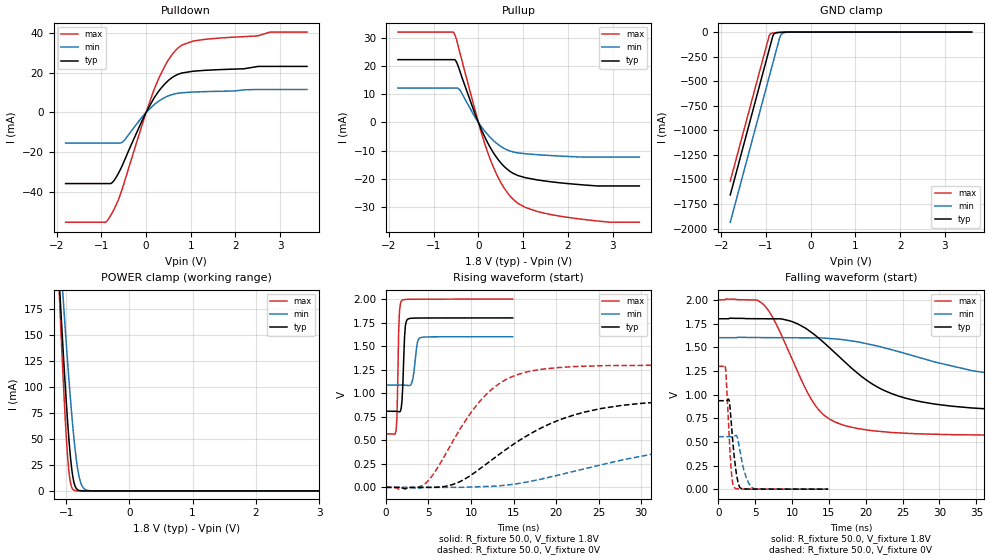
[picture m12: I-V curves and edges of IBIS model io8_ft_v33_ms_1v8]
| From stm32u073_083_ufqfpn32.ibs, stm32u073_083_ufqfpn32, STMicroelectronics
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[Model]   io8_ft_v33_ms_1v8
Model_type I/O
Polarity   Non-Inverting
Enable   Active-Low
| CAP_THRESHOLD on pad IOFT is "UDTCAPC" :
| Rising=30.0% of vddiom   Falling=70.0% of vddiom
| C_comp min and max val. don't necessarily correlate with the min and max pvt
| but are the smallest and greatest pad capacitance found.
| var   typ   min   max
C_comp   2.10717pF  2.10454pF  2.16860pF
|C_comp_pullup   1.19920pF  1.17990pF  1.18495pF
|C_comp_pulldown   907.97820fF  924.64068fF  983.64502fF
Vinl = 480.0mV
Vinh = 1.4V
Vmeas = 900.0mV   | Reference voltage for timing measurements
Cref  = 50.0pF   | Timing specification test load capacitance value
Rref  = 100.0MOhm   | Timing specification test load resistance value
Vref  = 900.0mV   | Timing specification test load voltage
[Model Spec]
| TIME_THRESHOLD on pin ZIV33M is "CMOS" :
| Rising=50.0% of vddiom   Falling=50.0% of vddiom
Vinl 728.70000mV 655.70000mV 817.70000mV
Vinh 1.06430V 949.30000mV 1.16330V
| variable   typ   min   max
[Temperature Range] 25.0 140.0 -40.0
| variable   typ   min   max
[Voltage Range] 1.8V 1.6V 2.0V
| variable   typ   min   max
[POWER Clamp Reference] 1.8V 1.6V 2.0V
| variable   typ   min   max
[GND Clamp Reference] 0V 0V 0V
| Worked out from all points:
|   slope of the pulldown table from 0 to 0.27 V, typ, clamps not added: 26.3 ohm
|   slope of the pullup table from 0 to 0.27 V, typ, clamps not added: 30 ohm
|   GND clamp passes 1 mA (typ) near -0.61 V on its own axis
|   POWER clamp passes 1 mA (typ) near -0.81 V on its own axis
|   rising waveform, R_fixture 50.0, V_fixture 1.8V: 20-80 % time 251ps typ, 394ps min, 200ps max; typ from 0.809 V to 1.8 V
|   falling waveform, R_fixture 50.0, V_fixture 1.8V: 20-80 % time 10.1ns typ, 18ns min, 5.4ns max; typ from 1.8 V to 0.809 V
|   rising waveform, R_fixture 50.0, V_fixture 0V: 20-80 % time 10.5ns typ, 18.9ns min, 5.99ns max; typ from 0 V to 0.935 V
|   falling waveform, R_fixture 50.0, V_fixture 0V: 20-80 % time 695ps typ, 1.01ns min, 535ps max; typ from 0.935 V to 0 V
[POWER Clamp]
-1.8V     1.053A     943.1mA    1.262A
-1.11V    202.2mA    242.3mA    190.9mA
-1.09V    180mA      223.6mA    163.4mA
-1.05V    136.9mA    187mA      110.9mA
-980mV    68.91mA    126.1mA    35.23mA
-940mV    37.57mA    94.11mA    10.65mA
-880mV    8.969mA    52.17mA    807.4uA
-830mV    1.697mA    25.82mA    75.79uA
-790mV    394.2uA    12.22mA    11.25uA
-740mV    61.25uA    3.879mA    1.034uA
-660mV    3.073uA    483.4uA    22.7nA
3.6V      0A         0A         0A
[GND Clamp]
-1.8V     -1.658A    -1.935A    -1.517A
-930mV    -179mA     -456mA     -38.91mA
-900mV    -128mA     -405mA     -17.65mA
-850mV    -44.09mA   -320mA     -9.519mA
-830mV    -24.74mA   -286mA     -8.302mA
-790mV    -9.695mA   -218mA     -6.49mA
-700mV    -2.938mA   -65mA      -3.294mA
-670mV    -2.157mA   -31.85mA   -2.435mA
-640mV    -1.545mA   -16.21mA   -1.699mA
-570mV    -571.9uA   -3.807mA   -536.5uA
-420mV    -14.26uA   -143.3uA   -5.434uA
3.6V      449.1pA    102.3nA    316.4pA
| variable   typ   min   max
[Pullup Reference] 1.8V 1.6V 2.0V
| variable   typ   min   max
[Pulldown Reference] 0V 0V 0V
[Pullup]
-1.8V     22.25mA    12.18mA    32.02mA
-550mV    22.25mA    12.18mA    31.76mA
-500mV    21.67mA    12.18mA    29.82mA
-420mV    18.45mA    11.57mA    25.1mA
-90mV     3.62mA     2.224mA    5.223mA
240mV     -8.143mA   -4.875mA   -12mA
540mV     -15mA      -8.867mA   -22.31mA
870mV     -18.72mA   -10.75mA   -28.48mA
1.33V     -20.4mA    -11.44mA   -31.6mA
1.9V      -21.5mA    -11.96mA   -33.39mA
2.94V     -22.49mA   -12.26mA   -35.33mA
3.6V      -22.49mA   -12.26mA   -35.33mA
[Pulldown]
-1.8V     -35.76mA   -15.41mA   -55.17mA
-910mV    -35.76mA   -15.41mA   -55.17mA
-830mV    -35.76mA   -15.41mA   -53.18mA
-710mV    -34mA      -15.41mA   -48.42mA
-520mV    -26.05mA   -14.75mA   -37.5mA
-90mV     -4.145mA   -2.306mA   -6.327mA
230mV     8.974mA    4.797mA    14.24mA
490mV     15.87mA    8.223mA    26.01mA
750mV     19.43mA    9.743mA    33.01mA
1.33V     21.16mA    10.45mA    36.75mA
2.78V     23.13mA    11.52mA    40.36mA
3.6V      23.13mA    11.52mA    40.37mA
[Ramp]
dV/dt_r 560.73538mV/10.49232ns 332.40859mV/18.92225ns 778.78175mV/5.99118ns
dV/dt_f 594.8441mV/10.08343ns 308.2854mV/17.96303ns 859.13306mV/5.40114ns
R_load = 50.0
| Removed startup time: 0s 0s 0s  .
| Removed end time: 14.9ns.
[Rising Waveform]
R_fixture   = 50.0
V_fixture   = 1.8V
V_fixture_min = 1.6V
V_fixture_max = 2.0V
0s        808.6mV    1.086V     568.1mV
1.2ns     808.3mV    1.086V     602.5mV
1.3ns     807.6mV    1.086V     728.9mV
1.5ns     803.8mV    1.086V     1.641V
1.6ns     801.6mV    1.086V     1.871V
1.9ns     923.4mV    1.086V     1.987V
2.2ns     1.607V     1.085V     1.995V
2.6ns     1.788V     1.082V     1.997V
4ns       1.799V     1.587V     1.998V
14.9ns    1.8V       1.6V       2V
| Removed startup time: 0s 0s 0s  .
| Removed end time: 199.9ns.
[Falling Waveform]
R_fixture   = 50.0
V_fixture   = 1.8V
V_fixture_min = 1.6V
V_fixture_max = 2.0V
0s        1.8V       1.6V       2V
6.3ns     1.8V       1.601V     1.939V
7.8ns     1.8V       1.6V       1.754V
12.3ns    1.675V     1.6V       993.5mV
14.6ns    1.529V     1.595V     766.5mV
19.5ns    1.187V     1.547V     633.4mV
23.4ns    1.013V     1.476V     599.3mV
38.3ns    840.1mV    1.206V     570.7mV
52.9ns    814.4mV    1.126V     568.3mV
199.9ns   808.6mV    1.086V     568.1mV
| Removed startup time: 0s 0s 0s  .
| Removed end time: 199.9ns.
[Rising Waveform]
R_fixture   = 50.0
V_fixture   = 0V
V_fixture_min = 0V
V_fixture_max = 0V
0s        -9.641uV   -5.549uV   -9.62uV
4.8ns     -271.2uV   -459.8uV   54.1mV
8.5ns     51.82mV    101.8uV    586.6mV
10.8ns    180.5mV    5.891mV    887.9mV
13.2ns    342.8mV    15.15mV    1.094V
20.1ns    705.8mV    126.3mV    1.271V
30.3ns    893.8mV    335.8mV    1.296V
40.3ns    927.2mV    462.2mV    1.298V
54.8ns    933.9mV    530.6mV    1.298V
199.9ns   934.6mV    554mV      1.298V
| Removed startup time: 0s 0s 0s  .
| Removed end time: 14.9ns.
[Falling Waveform]
R_fixture   = 50.0
V_fixture   = 0V
V_fixture_min = 0V
V_fixture_max = 0V
0s        934.6mV    554mV      1.298V
1ns       933.9mV    554mV      1.276V
1.5ns     935.2mV    553.7mV    528mV
1.7ns     776.7mV    553.5mV    272.4mV
1.9ns     575.3mV    553.8mV    93.87mV
2.2ns     324.8mV    560.1mV    14.97mV
2.9ns     22.12mV    422.1mV    2.394mV
3.6ns     2.47mV     170.3mV    1.549mV
4.6ns     1.047mV    15.09mV    1.204mV
14.9ns    285.7uV    305.6uV    145.1uV
